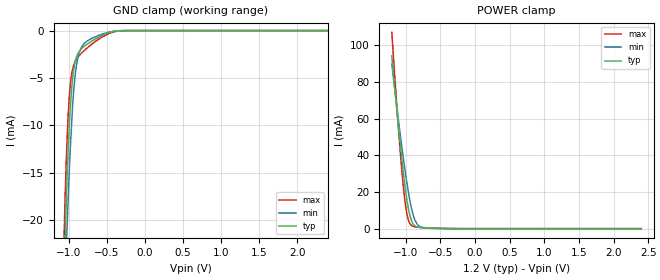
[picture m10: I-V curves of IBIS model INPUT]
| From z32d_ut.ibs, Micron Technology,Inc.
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| MODEL INPUT (Add/Cmd/Ctrl Input Model, 1600-3200Mbps)
[Model]   INPUT
Model_type   Input
Vinl = 510.000mV
Vinh = 690.000mV
|   typ   min   max
|C_comp   0.362pF   0.312pF   0.412pF
C_comp_power_clamp   0.181pF   0.156pF   0.206pF
C_comp_gnd_clamp   0.181pF   0.156pF   0.206pF
[Model Spec]
| Input threshold voltage corners
Vinl   0.5100V   0.4800V   0.5400V
Vinh   0.6900V   0.6600V   0.7200V
| Dynamic Overshoot Parameters from DDR4 Specification
|D_overshoot_ampl_h   0.30   NA   NA
|D_overshoot_ampl_l   0.30   NA   NA
|D_overshoot_area_h   0.1754n   NA   NA
|D_overshoot_area_l   0.1762n   NA   NA
[Receiver Thresholds]
Vth   =  0.600V
Vth_min  =  0.5880V
Vth_max  =  0.6120V
Vinh_ac  =  0.090V
Vinh_dc  =  0.065V
Vinl_ac  = -0.090V
Vinl_dc  = -0.065V
Tslew_ac =  5.000ns |Not specified, so set to high value
Threshold_sensitivity = 0.50
Reference_supply Power_clamp_ref
[Voltage Range]   1.2000V   1.1400V   1.2600V
[POWER Clamp Reference]   1.2000V   1.1400V   1.2600V
| Junction Temperature (Ambient temp is 35C typ, 125C min, -40C max)
[Temperature Range]   50.0   140.0   -40.0
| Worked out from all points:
|   GND clamp passes 1 mA (typ) near -0.68 V on its own axis
|   POWER clamp passes 1 mA (typ) near -0.84 V on its own axis
[GND Clamp]
|   Voltage   I(typ)   I(min)   I(max)
-1.2V     -75.7mA    -73.15mA   -81.94mA
-1.06V    -25.47mA   -30.15mA   -21.29mA
-1.045V   -21.28mA   -26.41mA   -16.8mA
-1.025V   -16.24mA   -21.42mA   -12.02mA
-1.01V    -13.04mA   -18.29mA   -9.212mA
-980mV    -8.049mA   -12.51mA   -5.739mA
-950mV    -5.074mA   -7.962mA   -4.107mA
-920mV    -3.415mA   -5.011mA   -3.338mA
-865mV    -2.23mA    -2.372mA   -2.662mA
-775mV    -1.523mA   -1.197mA   -1.95mA
-315mV    -13.35uA   -11.28uA   -18.46uA
2.4V      0A         0A         0A
[POWER Clamp]
|   Voltage   I(typ)   I(min)   I(max)
-1.2V     94.24mA    89.76mA    107mA
-1.1V     54.19mA    57.92mA    52.68mA
-1.065V   41.3mA     47.43mA    35.99mA
-1.03V    29.43mA    37.45mA    21.62mA
-995mV    19.04mA    28.15mA    10.83mA
-975mV    14.08mA    23.29mA    6.744mA
-940mV    7.306mA    15.46mA    2.843mA
-910mV    3.836mA    10.08mA    1.58mA
-870mV    1.616mA    5.02mA     1.03mA
-830mV    856.5uA    2.219mA    837.6uA
-700mV    369.3uA    304.1uA    508.7uA
2.4V      0A         0A         0A
